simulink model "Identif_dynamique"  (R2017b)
settings: Solver=ode5  StartTime=0.0  StopTime=inf  FixedStep=0.005  RelTol=1e-3  AbsTol=1e-6
undefined symbols (not defined in the file or in its folder): RTDAC4PCIBaseAddress

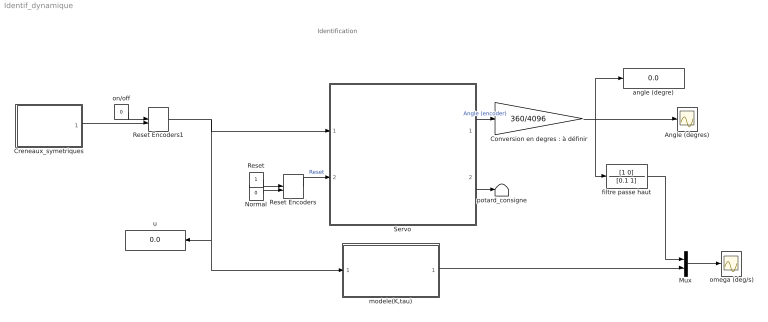
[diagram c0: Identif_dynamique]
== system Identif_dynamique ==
  note: Identification
  " omega (deg/s)" : Scope
  Angle (degres) : Scope
  "Conversion en degres : à définir" : Gain  Gain=360/4096
  Creneaux_symetriques : Subsystem
  Mux : Mux  Inputs=2
  Normal : Constant  Value=0
  Reset : Constant
  Reset Encoders : ManualSwitch  CurrentSetting=0
  Reset Encoders1 : ManualSwitch  CurrentSetting=0
  Servo : Subsystem  mask{BaseAddress=RTDAC4PCIBaseAddress(-1,-1), T0=0.005}
      mask prompts: BaseAddress "Base Address:"; T0 "Sampling Period:"
  angle (degre) : Display
  filtre passe haut : TransferFcn  Numerator=[1 0]  Denominator=[0.1 1]
  modele(K,tau) : Subsystem
  on/off : Constant  Value=0
  potard_consigne : Terminator
  u : Display
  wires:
  Reset Encoders/1 -> Servo/2(Reset Encoder)  "Reset"
  Normal/1 -> Reset Encoders/2
  Reset/1 -> Reset Encoders/1
  Servo/2(Set-up) -> potard_consigne/1
  Servo/1(Codeur_angulaire) -> "Conversion en degres : à définir"/1  "Angle (encoder)"
  "Conversion en degres : à définir"/1 -> Angle (degres)/1, angle (degre)/1, filtre passe haut/1
  filtre passe haut/1 -> Mux/1
  modele(K,tau)/1(thetapoint) -> Mux/2
  Mux/1 -> " omega (deg/s)"/1
  on/off/1 -> Reset Encoders1/1
  Reset Encoders1/1 -> modele(K,tau)/1(u), u/1, Servo/1(PWM Control)
  Creneaux_symetriques/1(u) -> Reset Encoders1/2

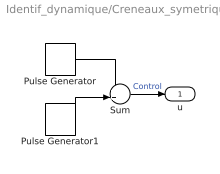
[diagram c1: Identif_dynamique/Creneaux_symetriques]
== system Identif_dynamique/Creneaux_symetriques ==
  Pulse Generator : DiscretePulseGenerator  PulseType=Time based  Amplitude=0.6  Period=0.005*floor(15/0.005)  PulseWidth=50  PhaseDelay=0.005*floor(0*15/0.005/4)
  Pulse Generator1 : DiscretePulseGenerator  PulseType=Time based  Amplitude=-0.6  Period=0.005*floor(15/0.005)  PulseWidth=50  PhaseDelay=0.005*floor(2*15/0.005/4)
  Sum : Sum
  u : Outport
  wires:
  Pulse Generator/1 -> Sum/1
  Pulse Generator1/1 -> Sum/2
  Sum/1 -> u/1  "Control"

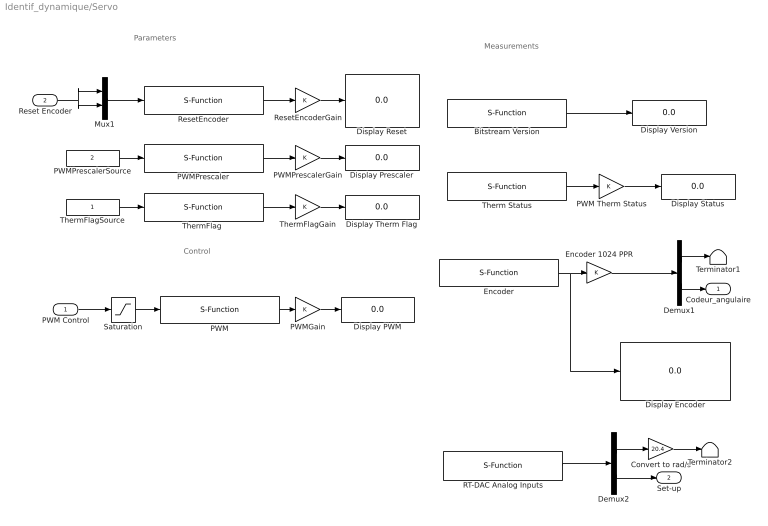
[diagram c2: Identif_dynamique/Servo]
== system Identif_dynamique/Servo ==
  note: Parameters
  note: Control
  note: Measurements
  PWM Control : Inport
  Reset Encoder : Inport  Port=2
  Bitstream Version : S-Function  FunctionName=Servo_BitstreamVersion  Parameters=BaseAddress, T0  SFunctionDeploymentMode=off  EnableBusSupport=off
  Convert to rad/s : Gain  Gain=20.4
  Demux1 : Demux  Outputs=2
  Demux2 : Demux  Outputs=2
  Display Encoder : Display
  Display PWM : Display
  Display Prescaler : Display
  Display Reset : Display
  Display Status : Display
  Display Therm Flag : Display
  Display Version : Display
  Encoder : S-Function  FunctionName=Servo_Encoder  Parameters=BaseAddress, T0  SFunctionDeploymentMode=off  EnableBusSupport=off
  Encoder 1024 PPR : Gain
  Mux1 : Mux  Inputs=2
  PWM : S-Function  FunctionName=Servo_PWM  Parameters=BaseAddress, T0  SFunctionDeploymentMode=off  EnableBusSupport=off
  PWM Therm Status : Gain
  PWMGain : Gain
  PWMPrescaler : S-Function  FunctionName=Servo_PWMPrescaler  Parameters=BaseAddress, T0  SFunctionDeploymentMode=off  EnableBusSupport=off
  PWMPrescalerGain : Gain
  PWMPrescalerSource : Constant  Value=2
  RT-DAC Analog Inputs : S-Function  FunctionName=servo_analoginputs  Parameters=BaseAddress, [1 0], [1 1], T0  SFunctionDeploymentMode=off  EnableBusSupport=off
  ResetEncoder : S-Function  FunctionName=Servo_ResetEncoder  Parameters=BaseAddress, T0  SFunctionDeploymentMode=off  EnableBusSupport=off
  ResetEncoderGain : Gain
  Saturation : Saturate  UpperLimit=1  LowerLimit=-1
  Terminator1 : Terminator
  Terminator2 : Terminator
  Therm Status : S-Function  FunctionName=Servo_PWMTherm  Parameters=BaseAddress, T0  SFunctionDeploymentMode=off  EnableBusSupport=off
  "ThermFlag " : S-Function  FunctionName=Servo_ThermFlag  Parameters=BaseAddress, T0  SFunctionDeploymentMode=off  EnableBusSupport=off
  ThermFlagGain : Gain
  ThermFlagSource : Constant
  Codeur_angulaire : Outport
  Set-up : Outport  Port=2
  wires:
  Encoder/1 -> Encoder 1024 PPR/1, Display Encoder/1
  Saturation/1 -> PWM/1
  PWM/1 -> PWMGain/1
  PWMGain/1 -> Display PWM/1
  ResetEncoder/1 -> ResetEncoderGain/1
  PWMPrescaler/1 -> PWMPrescalerGain/1
  Mux1/1 -> ResetEncoder/1
  PWMPrescalerSource/1 -> PWMPrescaler/1
  ResetEncoderGain/1 -> Display Reset/1
  PWMPrescalerGain/1 -> Display Prescaler/1
  PWM Control/1 -> Saturation/1
  Encoder 1024 PPR/1 -> Demux1/1
  Therm Status/1 -> PWM Therm Status/1
  PWM Therm Status/1 -> Display Status/1
  Bitstream Version/1 -> Display Version/1
  Reset Encoder/1 -> Mux1/1, Mux1/2
  "ThermFlag "/1 -> ThermFlagGain/1
  ThermFlagSource/1 -> "ThermFlag "/1
  ThermFlagGain/1 -> Display Therm Flag/1
  Demux1/1 -> Terminator1/1
  Demux1/2 -> Codeur_angulaire/1
  RT-DAC Analog Inputs/1 -> Demux2/1
  Demux2/2 -> Set-up/1
  Demux2/1 -> Convert to rad/s/1
  Convert to rad/s/1 -> Terminator2/1

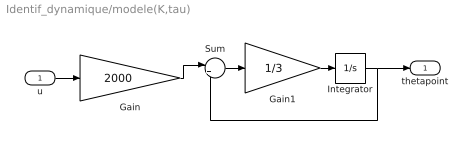
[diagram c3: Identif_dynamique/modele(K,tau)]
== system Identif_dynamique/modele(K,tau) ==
  u : Inport
  Gain : Gain  Gain=2000
  Gain1 : Gain  Gain=1/3
  Integrator : Integrator
  Sum : Sum  Inputs=|+-
  thetapoint : Outport
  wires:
  Gain/1 -> Sum/1
  Gain1/1 -> Integrator/1
  Integrator/1 -> thetapoint/1, Sum/2
  Sum/1 -> Gain1/1
  u/1 -> Gain/1
